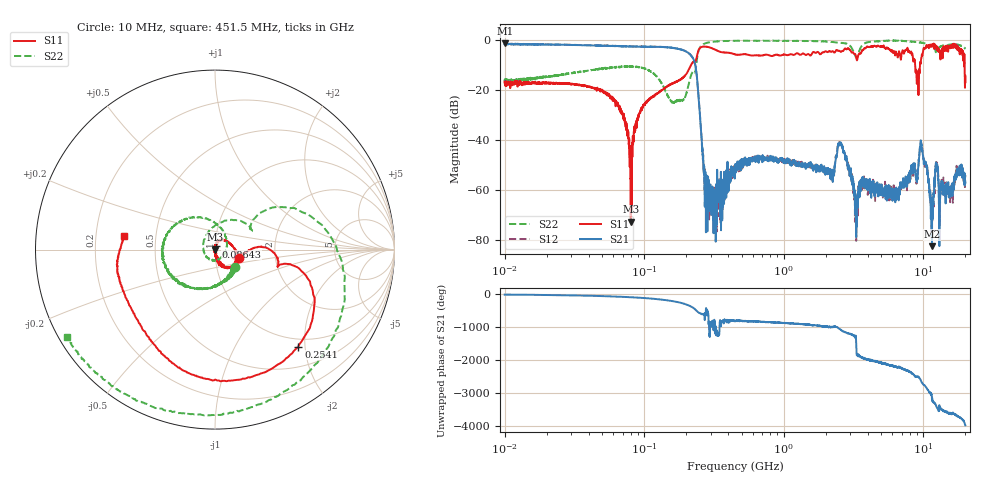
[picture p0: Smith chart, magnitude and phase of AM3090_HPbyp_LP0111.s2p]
# Hz S DB R 50
!freq MagS11 AngS11 MagS21 AngS21 MagS12 AngS12 MagS22 AngS22
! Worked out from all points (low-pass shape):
!   3201 points, 10 MHz to 20 GHz, reference 50 ohm
!   highest |S21| = -1.30 dB at 10.05 MHz (marker M1); lowest = -82.5 dB at 11.53 GHz (marker M2)
!   |S21| within 3 dB of the highest: start of sweep to 193.6 MHz
!   lowest |S11| = -72.7 dB at 80.1 MHz (marker M3), VSWR 1.00, Z = 50 + j0.0215 ohm
!   |S11| at or under -10 dB: start of sweep to 216.6 MHz; 8.726 GHz to 9.454 GHz (727.2 MHz wide, 8 % of centre); 19.73 GHz to end of sweep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
!   |S22| runs from -25.2 to -0.2 dB; largest |S21 - S12| = 0.042
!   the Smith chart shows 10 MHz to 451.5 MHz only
!   S11 on the Smith chart (normalised r, x): 10 MHz: 1.30, -0.13; 86.43 MHz: 1.01, +0.03; 254.1 MHz: 0.85, -1.87; 451.5 MHz: 0.33, +0.07
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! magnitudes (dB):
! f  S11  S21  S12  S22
! 10 MHz  -17.0  -1.8  -1.6  -16.4
! 10.05 MHz  -17.0  -1.3  -1.7  -17.7
! 35.55 MHz  -18.1  -2.1  -2.1  -12.7
! 64.08 MHz  -25.6  -2.4  -2.4  -11.0
! 80.1 MHz  -72.7  -2.6  -2.5  -10.8
! 86.43 MHz  -35.0  -2.6  -2.6  -10.8
! 126.1 MHz  -21.3  -2.8  -2.8  -15.3
! 163.7 MHz  -17.1  -3.3  -3.2  -25.1
! 221.9 MHz  -9.0  -7.0  -7.0  -12.8
! 254.1 MHz  -2.9  -34.7  -34.0  -2.6
! 287.5 MHz  -2.9  -57.4  -68.6  -1.1
! 447.2 MHz  -5.7  -51.4  -51.9  -0.3
! 451.5 MHz  -5.8  -53.1  -51.6  -0.4
! 1.59 GHz  -5.5  -50.3  -50.5  -0.4
! 2.222 GHz  -4.5  -53.0  -53.2  -0.8
! 2.533 GHz  -4.6  -41.0  -41.7  -1.1
! 3.273 GHz  -6.1  -65.1  -66.2  -6.9
! 5.639 GHz  -3.6  -58.1  -60.4  -0.3
! 9.692 GHz  -7.1  -42.1  -41.5  -1.1
! 11.53 GHz  -1.9  -82.5  -72.9  -2.1
! 12.41 GHz  -2.5  -50.6  -49.9  -4.2
! 20 GHz  -14.3  -57.1  -54.0  -3.6
